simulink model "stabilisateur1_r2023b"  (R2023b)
settings: Solver=VariableStepAuto  StartTime=0.0  StopTime=10.0  RelTol=1e-3
libraries: spsMeanLib x1, simulink x1

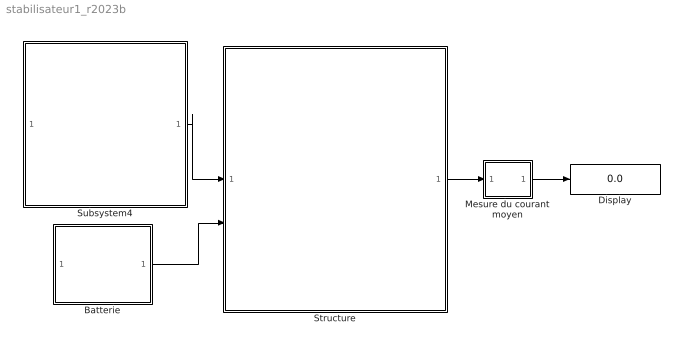
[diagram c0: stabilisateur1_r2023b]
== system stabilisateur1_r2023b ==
  Batterie : Subsystem  mask{unom=7.4}
      mask prompts: unom "Tension nominale (V)"
  Display : Display
  Mesure du courant moyen : Subsystem
  Structure : Subsystem
  Subsystem4 : Subsystem  mask{freq=0.5}
      mask prompts: freq "Fréquence (Hz)"
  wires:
  Batterie/1(Out1) -> Structure/2(In2)
  Structure/1(Out2) -> Mesure du courant moyen/1(In1)
  Mesure du courant moyen/1(Mean1) -> Display/1
  Subsystem4/1(Out1) -> Structure/1(In1)

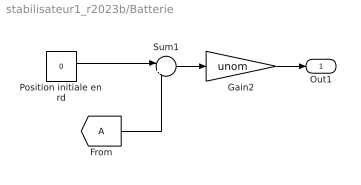
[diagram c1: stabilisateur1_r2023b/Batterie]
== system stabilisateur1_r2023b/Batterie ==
  From : From  TagVisibility=global
  Gain2 : Gain  Gain=unom
  Position initiale en rd : Constant  Value=0
  Sum1 : Sum  Inputs=|+-
  Out1 : Outport
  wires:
  Gain2/1 -> Out1/1
  Position initiale en rd/1 -> Sum1/1
  Sum1/1 -> Gain2/1
  From/1 -> Sum1/2

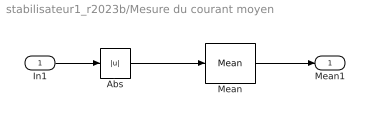
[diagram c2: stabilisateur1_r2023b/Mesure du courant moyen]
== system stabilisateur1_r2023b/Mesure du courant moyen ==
  In1 : Inport
  Abs : Abs
  Mean : spsMeanLib/Mean  Freq=60  Vinit=0  Ts=0
  Mean1 : Outport
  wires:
  Mean/1 -> Mean1/1
  In1/1 -> Abs/1
  Abs/1 -> Mean/1

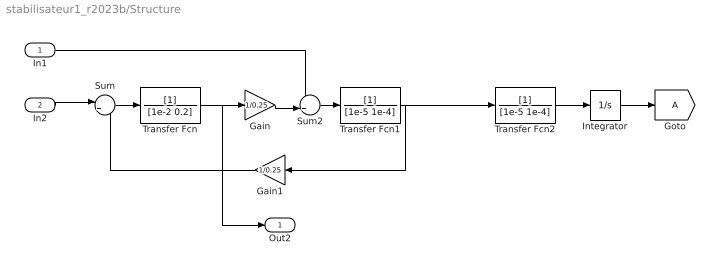
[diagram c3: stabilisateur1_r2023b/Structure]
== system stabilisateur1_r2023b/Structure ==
  In1 : Inport
  In2 : Inport  Port=2
  Gain : Gain  Gain=1/0.25
  Gain1 : Gain  Gain=1/0.25
  Goto : Goto  TagVisibility=global
  Integrator : Integrator
  Sum : Sum  Inputs=|+-
  Sum2 : Sum  Inputs=++|
  Transfer Fcn : TransferFcn  Denominator=[1e-2 0.2]
  Transfer Fcn1 : TransferFcn  Denominator=[1e-5 1e-4]
  Transfer Fcn2 : TransferFcn  Denominator=[1e-5 1e-4]
  Out2 : Outport
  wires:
  In2/1 -> Sum/1
  In1/1 -> Sum2/1
  Transfer Fcn/1 -> Out2/1, Gain/1
  Sum2/1 -> Transfer Fcn1/1
  Gain/1 -> Sum2/2
  Gain1/1 -> Sum/2
  Sum/1 -> Transfer Fcn/1
  Transfer Fcn1/1 -> Transfer Fcn2/1, Gain1/1
  Transfer Fcn2/1 -> Integrator/1
  Integrator/1 -> Goto/1

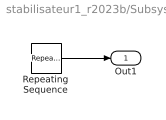
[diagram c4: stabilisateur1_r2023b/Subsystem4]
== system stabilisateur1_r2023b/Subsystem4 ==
  Repeating Sequence : simulink/Sources/Repeating Sequence  rep_seq_t=[0 1/freq 2/freq]  rep_seq_y=[0 1.5 0]
  Out1 : Outport
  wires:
  Repeating Sequence/1 -> Out1/1
